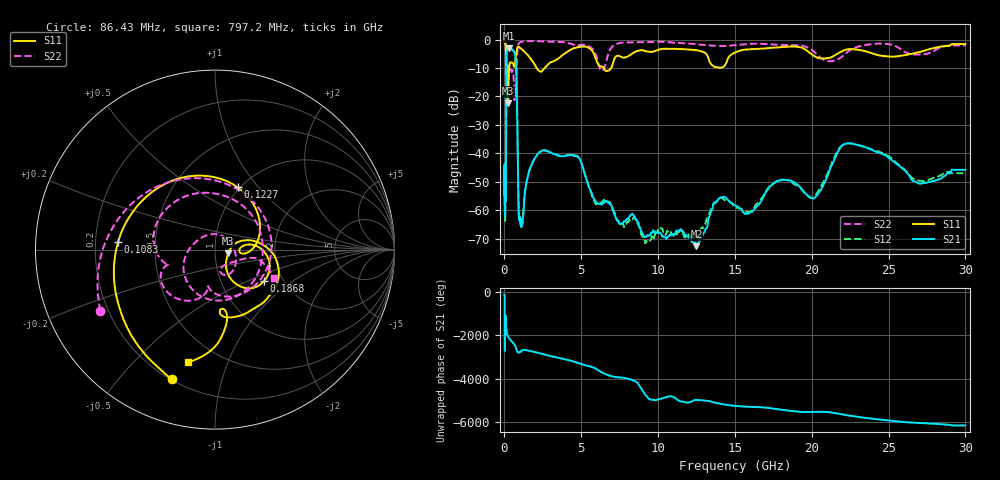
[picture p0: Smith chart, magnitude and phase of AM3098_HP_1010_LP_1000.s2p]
! Date/Time: Thu, Feb 28, 2019 8:42 AM
! Network Analyzer: Agilent Technologies E8364B Rev: A.07.50.67
! Sweep from 0.010 to 30.000 GHz, 1601 Points, Sweep Type: LOG
! Power Supply: 5.022 V, 0.002 A
# Hz S DB R 50
!freq MagS11 AngS11 MagS21 AngS21 MagS12 AngS12 MagS22 AngS22
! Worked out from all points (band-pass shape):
!   1601 points, 10 MHz to 30 GHz, reference 50 ohm
!   highest |S21| = -3.01 dB at 263.8 MHz (marker M1); lowest = -72.6 dB at 12.5 GHz (marker M2)
!   |S21| within 3 dB of the highest: 133.8 MHz to 706.7 MHz (572.9 MHz wide, 136 % of centre)
!   lowest |S11| = -22.4 dB at 242.3 MHz (marker M3), VSWR 1.16, Z = 57.8 - j2.46 ohm
!   |S11| at or under -10 dB: 191.5 MHz to 306.2 MHz (114.6 MHz wide, 46.1 % of centre); 2.094 GHz to 2.62 GHz (525.8 MHz wide, 22.3 % of centre); 6.467 GHz to 6.944 GHz (477.6 MHz wide, 7.12 % of centre)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
!   |S22| runs from -21.3 to -0.5 dB; largest |S21 - S12| = 0.0088
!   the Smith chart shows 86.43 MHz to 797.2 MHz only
!   S11 on the Smith chart (normalised r, x): 86.43 MHz: 0.20, -0.70; 108.3 MHz: 0.30, +0.04; 122.7 MHz: 0.97, +0.79; 186.8 MHz: 1.61, -0.63; 797.2 MHz: 0.34, -0.73
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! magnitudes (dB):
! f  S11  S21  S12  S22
! 10 MHz  -0.3  -44.7  -45.8  -0.6
! 38.04 MHz  -0.4  -58.9  -58.2  -0.9
! 48.85 MHz  -0.7  -50.3  -49.4  -1.2
! 86.43 MHz  -2.4  -55.1  -56.0  -2.8
! 108.3 MHz  -5.3  -30.4  -30.3  -6.8
! 122.7 MHz  -8.6  -11.6  -11.6  -10.2
! 144.7 MHz  -17.4  -4.6  -4.6  -13.5
! 186.8 MHz  -9.8  -3.6  -3.6  -9.0
! 242.3 MHz  -22.4  -3.0  -3.0  -11.3
! 263.8 MHz  -16.2  -3.0  -3.0  -10.8
! 550.5 MHz  -8.3  -3.9  -3.8  -11.0
! 655.8 MHz  -9.3  -4.5  -4.5  -21.3
! 797.2 MHz  -3.8  -15.6  -15.6  -8.8
! 959.3 MHz  -2.7  -63.2  -61.7  -1.2
! 2.084 GHz  -9.9  -40.8  -41.0  -0.6
! 4.71 GHz  -2.8  -41.0  -40.9  -2.1
! 7.926 GHz  -6.2  -63.3  -64.8  -1.0
! 12.5 GHz  -3.7  -72.6  -69.1  -1.7
! 14.09 GHz  -9.9  -55.6  -55.4  -2.3
! 20.1 GHz  -5.6  -55.9  -55.4  -4.1
! 22.56 GHz  -3.4  -36.5  -36.5  -3.5
! 30 GHz  -1.6  -45.7  -47.0  -2.1
